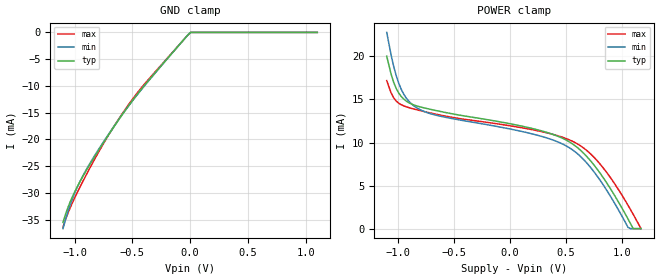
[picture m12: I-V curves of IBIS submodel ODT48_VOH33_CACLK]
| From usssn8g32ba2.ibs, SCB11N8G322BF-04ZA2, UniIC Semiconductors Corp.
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|   Submodel ODT48_VOH33_CACLK
[Submodel] ODT48_VOH33_CACLK
Submodel_type Dynamic_clamp
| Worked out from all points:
|   GND clamp passes 1 mA (typ) near -0.04 V on its own axis
[GND_clamp]
|Voltage   I(typ)   I(min)   I(max)
-1.1V     -35.54mA   -36.7mA    -36.41mA
-1.054V   -32.56mA   -33.29mA   -33.64mA
-1.031V   -31.34mA   -31.84mA   -32.46mA
-985mV    -29.22mA   -29.37mA   -30.32mA
-939mV    -27.35mA   -27.29mA   -28.32mA
-893mV    -25.62mA   -25.45mA   -26.4mA
-778mV    -21.58mA   -21.41mA   -21.85mA
-617mV    -16.31mA   -16.27mA   -16.17mA
-456mV    -11.54mA   -11.62mA   -11.28mA
-180mV    -4.474mA   -4.487mA   -4.391mA
4mV       0A         0A         0A
1.1V      0A         0A         0A
[POWER_clamp]
|Voltage   I(typ)   I(min)   I(max)
-1.1V     20.02mA    22.79mA    17.19mA
-1.039V   17.02mA    18.89mA    15.21mA
-993mV    15.74mA    16.89mA    14.57mA
-924mV    14.8mA     15.13mA    14.14mA
-855mV    14.35mA    14.24mA    13.88mA
-648mV    13.68mA    13.14mA    13.26mA
226mV     11.55mA    10.91mA    11.42mA
571mV     9.726mA    9.031mA    10.06mA
801mV     6.507mA    5.687mA    7.553mA
1.054V    1.118mA    147.2uA    2.711mA
1.1V      0A         0A         1.666mA
1.17V     0A         0A         0A
